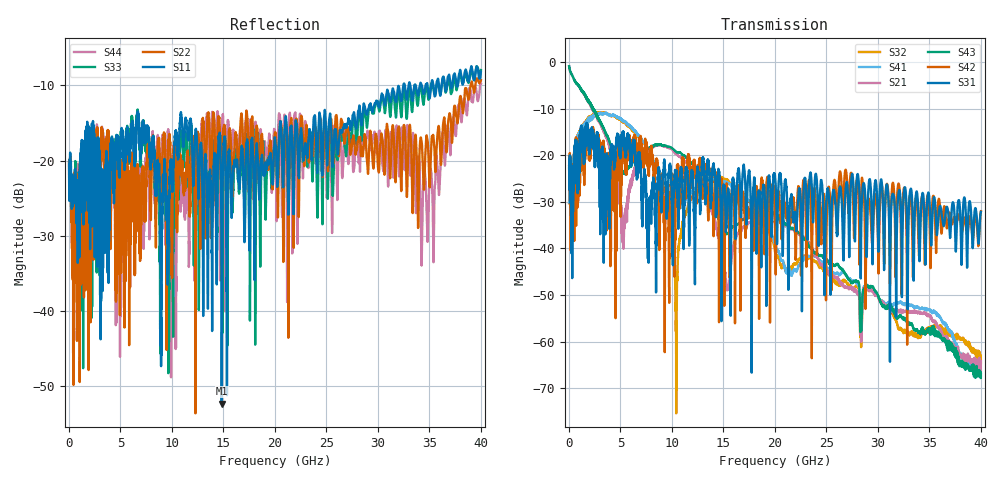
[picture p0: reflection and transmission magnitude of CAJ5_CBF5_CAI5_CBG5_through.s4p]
!Agilent Technologies,N5245A,MY49151062,A.09.90.19
!Agilent N5245A: A.09.90.19
!Date: Monday, October 10, 2016 09:29:31
!Correction: S11(Full 4 Port(1,2,3,4))
!S12(Full 4 Port(1,2,3,4))
!S13(Full 4 Port(1,2,3,4))
!S14(Full 4 Port(1,2,3,4))
!S21(Full 4 Port(1,2,3,4))
!S22(Full 4 Port(1,2,3,4))
!S23(Full 4 Port(1,2,3,4))
!S24(Full 4 Port(1,2,3,4))
!S31(Full 4 Port(1,2,3,4))
!S32(Full 4 Port(1,2,3,4))
!S33(Full 4 Port(1,2,3,4))
!S34(Full 4 Port(1,2,3,4))
!S41(Full 4 Port(1,2,3,4))
!S42(Full 4 Port(1,2,3,4))
!S43(Full 4 Port(1,2,3,4))
!S44(Full 4 Port(1,2,3,4))
!S4P File: Measurements: <S11,S12,S13,S14>,
!<S21,S22,S23,S24>,
!<S31,S32,S33,S34>,
!<S41,S42,S43,S44>:
# Hz S  RI  R 50
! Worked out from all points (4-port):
!   4000 points, 10 MHz to 40 GHz, reference 50 ohm
!   strongest paths, dB at 10 MHz, 10.01 GHz, 20.01 GHz, 30.01 GHz, 40 GHz:
!     S31: -22.8, -33.1, -24.8, -37.1, -32.1
!     S42: -22.3, -25.3, -37.8, -38.9, -32.0
!     S43: -0.8, -18.5, -32.7, -50.2, -67.0
!     S21: -0.9, -18.7, -33.3, -50.2, -64.2
!     S41: -30.1, -30.3, -38.9, -50.2, -67.5
!     S32: -30.3, -35.6, -40.8, -50.3, -64.6
!   lowest |S11| = -52.3 dB at 14.83 GHz (marker M1), VSWR 1.00, Z = 49.8 + j0.0362 ohm
!   |S11| at or under -10 dB: start of sweep to 32.47 GHz; 33.15 GHz to 33.56 GHz (410.1 MHz wide, 1.23 % of centre); 33.67 GHz to 34.08 GHz (408.1 MHz wide, 1.2 % of centre)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
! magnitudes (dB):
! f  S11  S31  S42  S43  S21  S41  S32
! 10 MHz  -20.5  -22.8  -22.3  -0.8  -0.9  -30.1  -30.3
! 5.88 GHz  -20.2  -18.6  -17.3  -22.5  -26.8  -13.5  -13.9
! 9.59 GHz  -36.5  -29.6  -28.6  -18.2  -18.3  -27.8  -30.4
! 10.42 GHz  -16.2  -24.4  -25.3  -19.3  -19.7  -30.8  -64.6
! 14.83 GHz  -52.3  -46.1  -25.8  -35.0  -40.6  -25.5  -24.7
! 34.27 GHz  -10.0  -29.0  -28.9  -57.6  -53.9  -52.8  -58.2
! 40 GHz  -8.2  -32.1  -32.0  -67.0  -64.2  -67.5  -64.6
